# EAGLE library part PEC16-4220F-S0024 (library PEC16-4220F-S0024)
Bourns Encoder 24ppr ppr 5 V dc Source: Datasheet
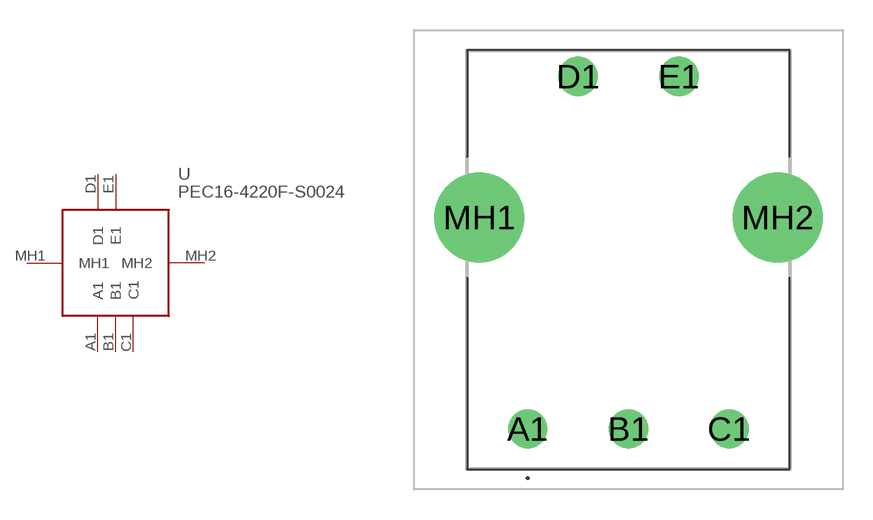
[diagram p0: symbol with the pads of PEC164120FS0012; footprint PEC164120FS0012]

Designator prefix U

## PEC16-4220F-S0024 (Arrow_Part_Number: PEC16-4220F-S0024; Arrow_Price-Stock: null?utm_currency=USD&region=nac; Description: Bourns Encoder 24ppr ppr 5 V dc; Height: 28mm; Manufacturer_Name: Bourns; Manufacturer_Part_Number: PEC16-4220F-S0024; Mouser_Part_Number: 652-PEC16-4220FS0024; Mouser_Price-Stock: https://www.mouser.co.uk/ProductDetail/Bourns/PEC16-4220F-S0024?qs=6FD5PBp7ZtQte%252Bg7b%2FiMUw%3D%3D)  [PEC164120FS0012]
A1  A1
B1  B1
C1  C1
D1  D1
E1  E1
MH1  MH1
MH2  MH2

## Footprint PEC164120FS0012 (pad centres in mm)
PEC16-4120F-S0012-1
drill 1.3 pad 1.95: A1 0,0; B1 5,0; C1 10,0; D1 2.5,17.5; E1 7.5,17.5
drill 2.973 pad 4.46: MH1 -2.4,10.5; MH2 12.4,10.5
